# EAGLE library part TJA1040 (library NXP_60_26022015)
High speed CAN transceiver The TJA1040 is the interface between the Controller Area Network (CAN) protocol controller and the physical bus. It is primarily intended for high speed applications, up to 1 MBaud, in passenger cars. The device provides differential transmit capability to the bus and differential receive capability to the CAN controller. The TJA1040 is the next step up from the TJA1050 high speed CAN transceiver. Being pin compatible and offering the same excellent EMC performance, the TJA1040 also features: An ideal passive behaviour when supply voltage is off A very low-current standby mode with remote wake-upcapability via the bus. This makes the TJA1040 an excellent choice in nodes which can be in power-down or standby mode in partially powered networks. AAL Eindhoven MK
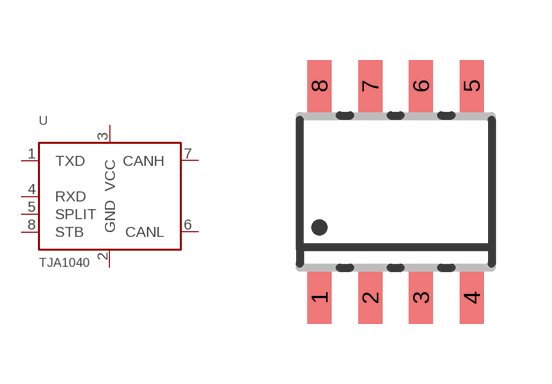
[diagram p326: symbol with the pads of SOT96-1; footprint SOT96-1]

Designator prefix U

## TJA1040T  [SOT96-1]
1  TXD  out
2  GND
3  VCC
4  RXD
5  SPLIT  pwr
6  CANL
7  CANH
8  STB  pas

## Footprint SOT96-1 (pad centres in mm)
SOT96-1 SO8: plastic small outline package; 8 leads; body width 3.9 mm JEDEC: MS-012 IEC: 076E03
smd 0.6 x 1.3: 1 -1.905,-2.65; 2 -0.635,-2.65; 3 0.635,-2.65; 4 1.905,-2.65; 5 1.905,2.65; 6 0.635,2.65; 7 -0.635,2.65; 8 -1.905,2.65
